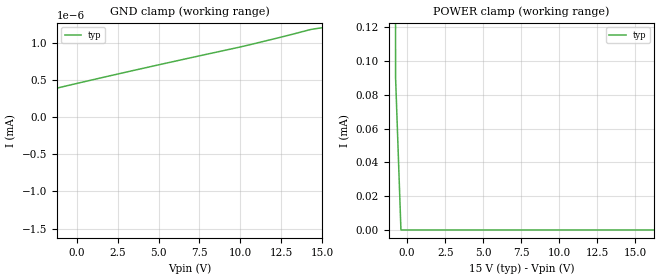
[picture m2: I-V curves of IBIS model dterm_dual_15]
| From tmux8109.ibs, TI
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| dterm_dual_15
[Model]   dterm_dual_15
Model_type   Terminator
|   typ   min   max
C_comp   6.362683e-12   NA   NA
[Voltage Range]   15   NA   NA
[Temperature Range]   27   NA   NA
[Power Clamp Reference]   15   NA   NA
[GND Clamp Reference]   0   NA   NA
[GND Clamp]
|   Voltage   I(typ)   I(min)   I(max)
-20V      -2.259A    NA         NA
-15.4V    -38.2nA    NA         NA
-15.05V   -269.4pA   NA         NA
-11.87V   -146pA     NA         NA
-9.04V    -16.46pA   NA         NA
1.566V    532.6pA    NA         NA
10.05V    946.3pA    NA         NA
14.29V    1.178nA    NA         NA
15V       1.202nA    NA         NA
[POWER Clamp]
|   Voltage   I(typ)   I(min)   I(max)
-5V       744mA      NA         NA
-1.111V   26.13mA    NA         NA
-757.6mV  90.5uA     NA         NA
-404mV    1.574nA    NA         NA
30V       -267.4pA   NA         NA
